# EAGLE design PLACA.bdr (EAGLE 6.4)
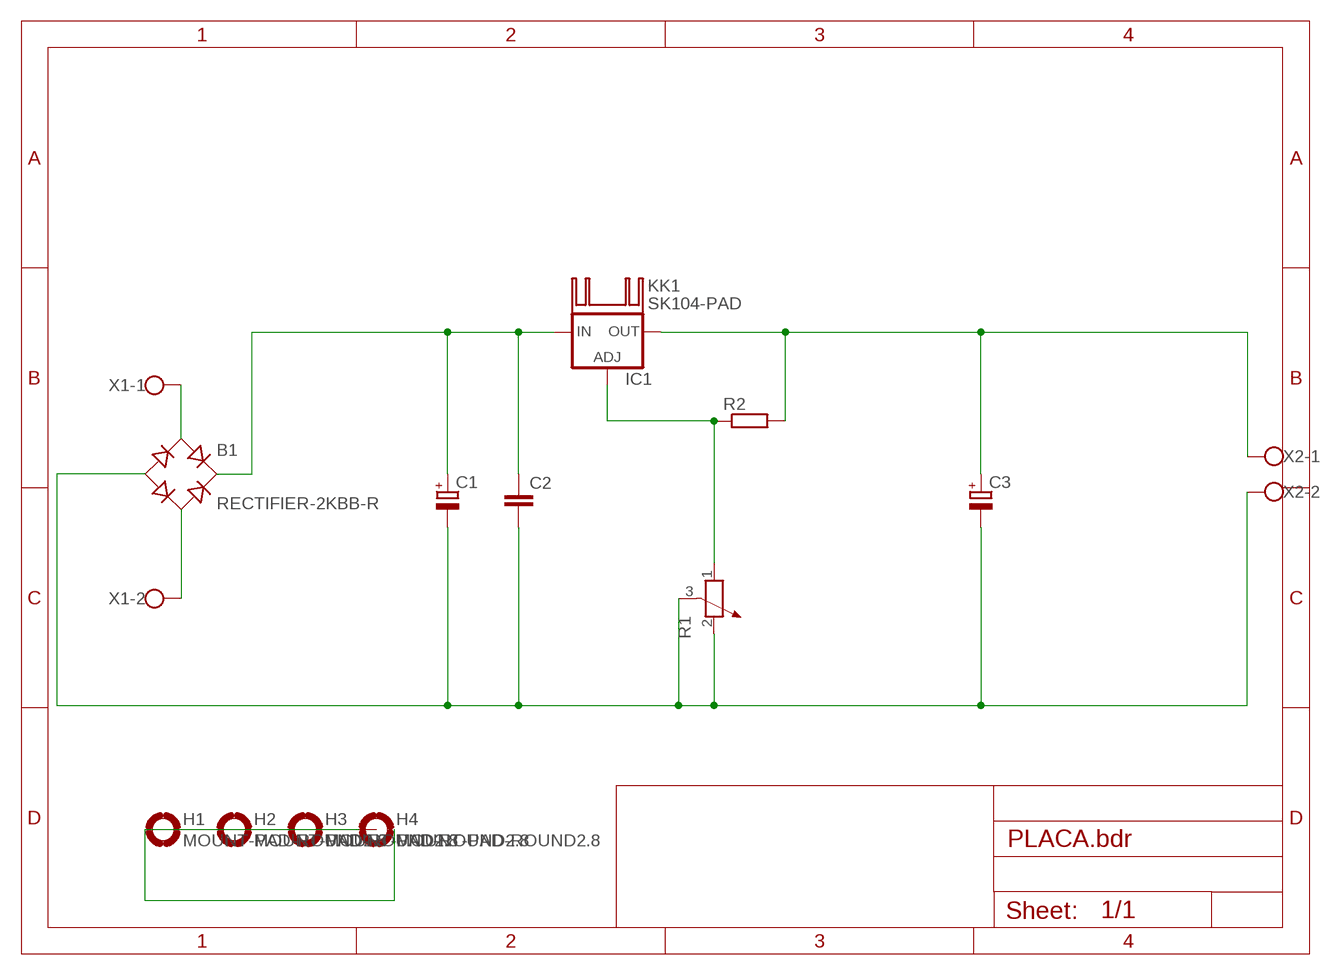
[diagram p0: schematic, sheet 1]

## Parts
B1  RECTIFIER-2KBB-R  [2KBB-R]
C1  CPOL-EUE7.5-16  [E7,5-16]
C2  C-EU050-025X075  [C050-025X075]
C3  CPOL-EUE2,5-6E  [E2,5-6E]
H1  MOUNT-PAD-ROUND2.8  [2,8-PAD]
H2  MOUNT-PAD-ROUND2.8  [2,8-PAD]
H3  MOUNT-PAD-ROUND2.8  [2,8-PAD]
H4  MOUNT-PAD-ROUND2.8  [2,8-PAD]
IC1  LM317TS  [317TS]
KK1  SK104-PAD  [SK104-PAD]
R1  POTENTIOMETER_PT-10  [PT-10]
R2  R-EU_0207/10  [0207/10]
X1  W237-102  [W237-102]
X2  W237-102  [W237-102]

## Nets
N$1: B1.AC1 X1.1
N$2: B1.AC2 X1.2
N$3: B1.- C1.- C2.2 C3.- R1.2 R1.3 X2.2
N$4: B1.+ C1.+ C2.1 IC1.3(IN)
N$5: C3.+ IC1.2(OUT) R2.2 X2.1
N$6: H1.B2,8(MOUNT) H2.B2,8(MOUNT) H3.B2,8(MOUNT) H4.B2,8(MOUNT)
N$7: IC1.1(ADJ) R1.1 R2.1
Unconnected: KK1.K1(K) KK1.K2(K)

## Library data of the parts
B1 = rectifier:RECTIFIER-: Rectifier
C1 C3 = rcl:CPOL-EU: POLARIZED CAPACITOR, European symbol
C2 = rcl:C-EU: CAPACITOR, European symbol
H1-H4 = holes:MOUNT-PAD-ROUND: MOUNTING PAD, round
IC1 = v-reg:LM317TS: VOLTAGE REGULATOR
KK1 = heatsink:SK104-PAD: HEATSINK
R1 = rcl:POTENTIOMETER_: Potentiometer
R2 = rcl:R-EU_: RESISTOR, European symbol
X1 X2 = con-wago-500:W237-102: WAGO SCREW CLAMP; MPN: 237-102; OC_FARNELL: unknown; OC_NEWARK: 70K9898

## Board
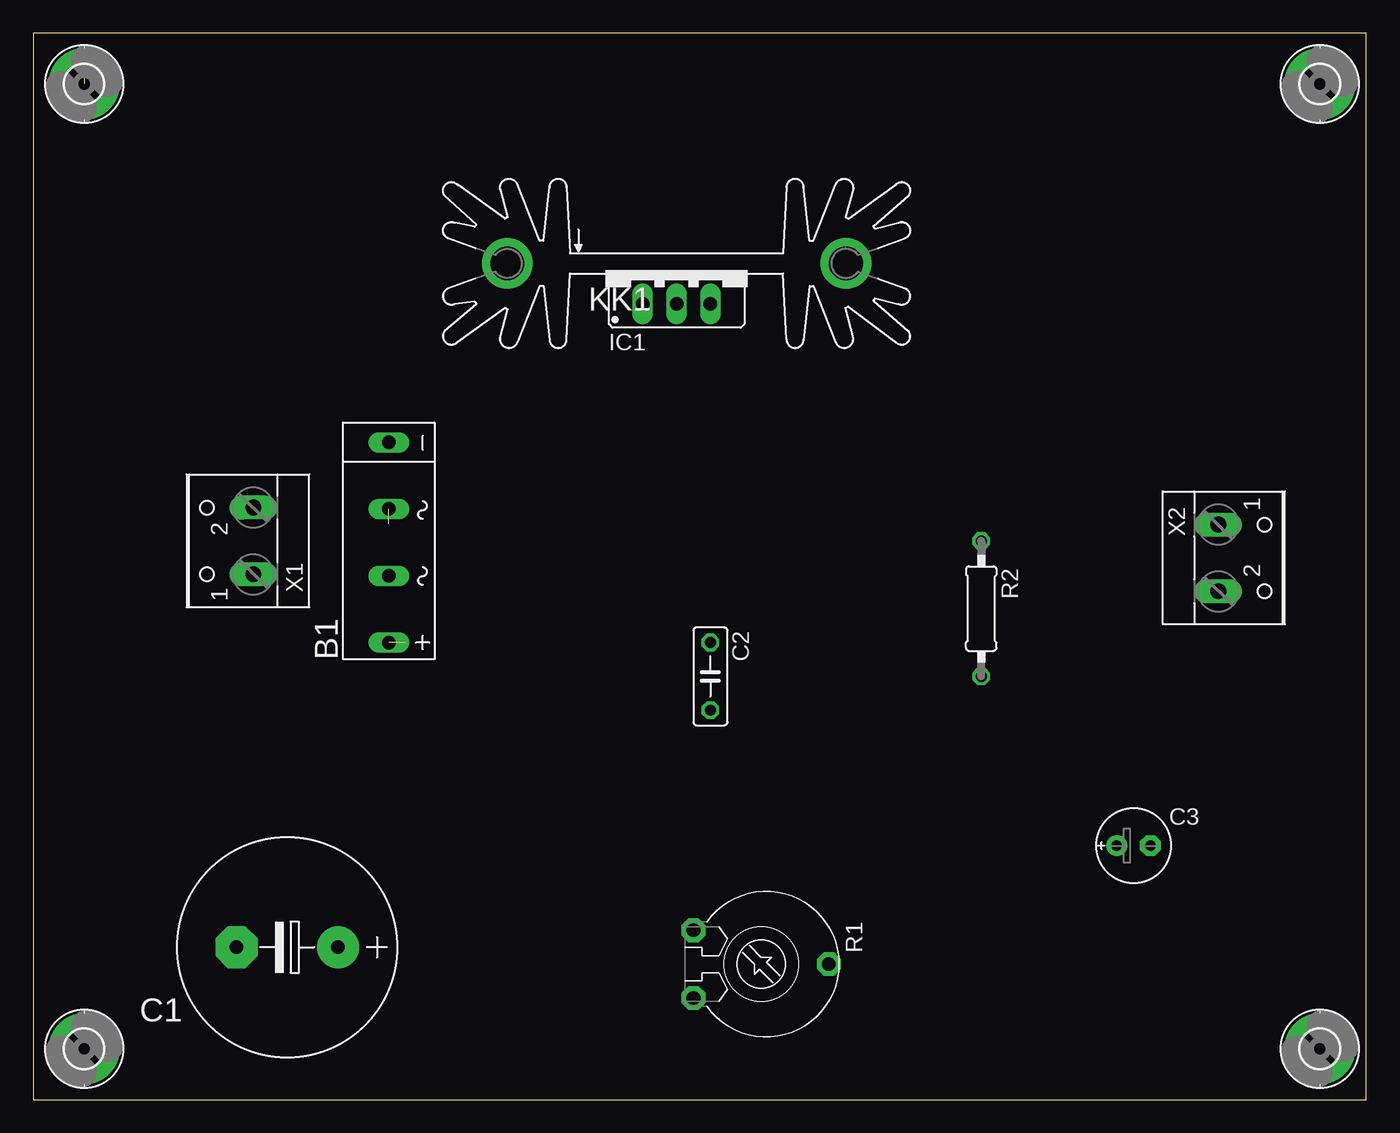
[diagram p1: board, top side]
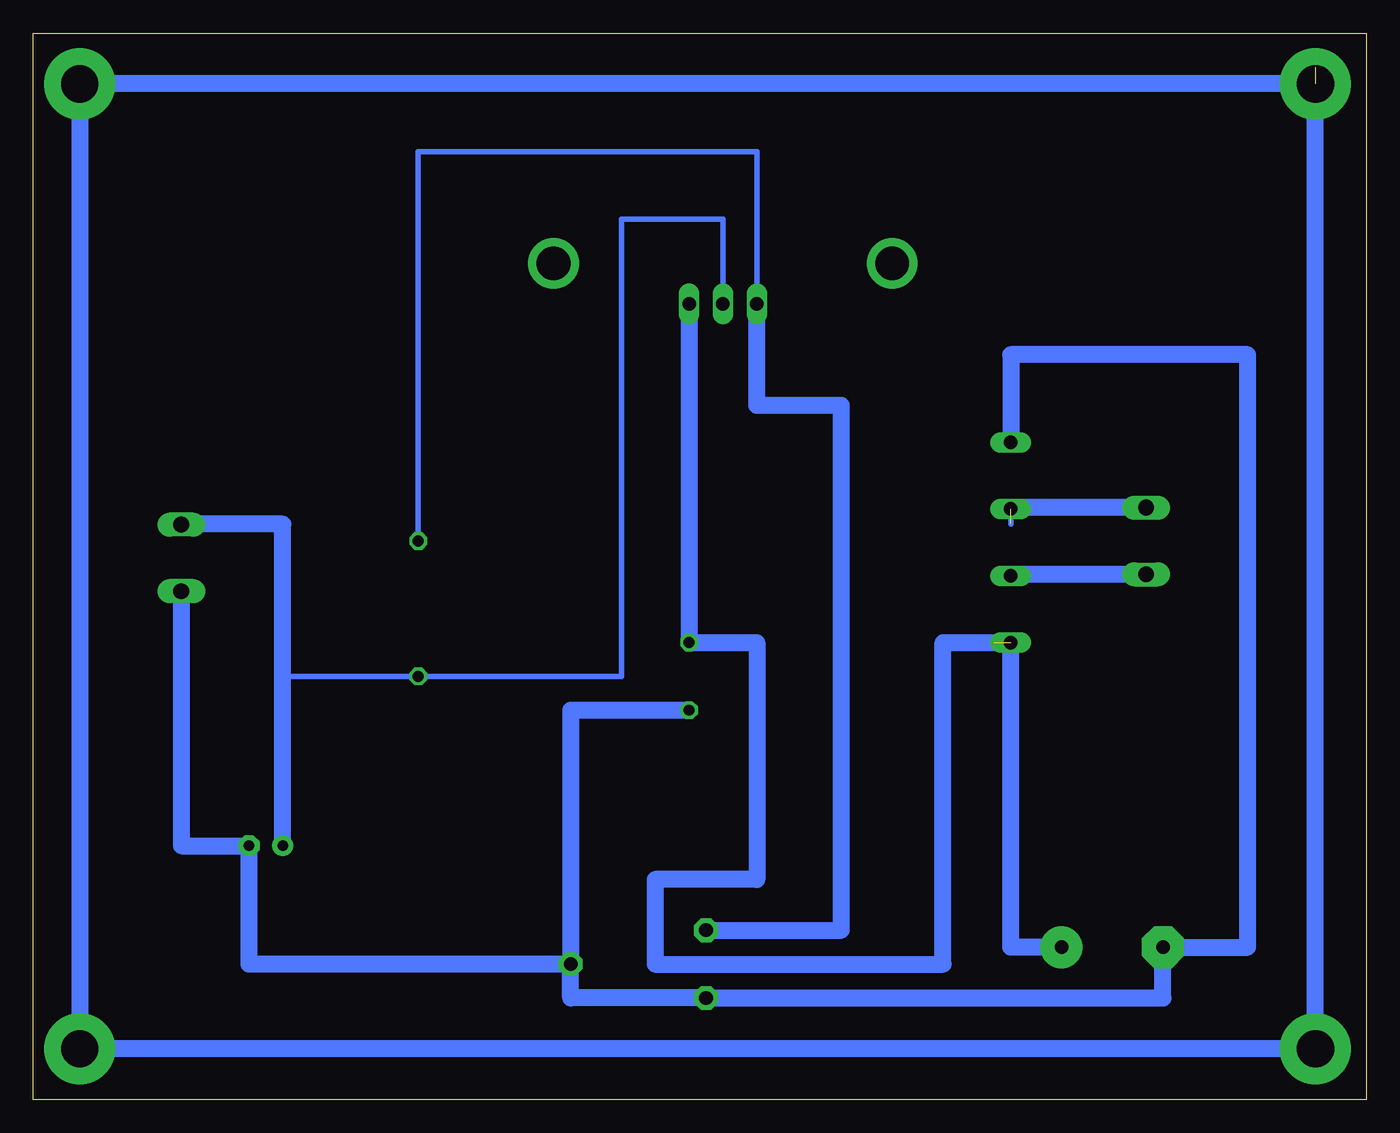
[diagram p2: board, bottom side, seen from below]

Size 100 x 80 mm. Coordinates in mm from the lower left corner, seen from the top.
Outline: 0,0 100,0 100,80 0,80 0,0
Copper layers (1*16): Top 0.035mm / dielectric 1.5mm / Bottom 0.035mm
Design rules "default": minimum track width 10mil, minimum drill 24mil, track to track 8mil, track to pad 8mil, pad to pad 8mil, via to via 8mil, smd to smd 8mil, copper to edge 40mil, drill to drill 8mil, minimum pad ring 10mil, minimum via ring 8mil, stop-mask expansion 4mil, vias tented up to drill 0mil, thermal gap 10mil

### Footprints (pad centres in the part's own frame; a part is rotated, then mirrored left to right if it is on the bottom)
2KBB-R = drill 1.016 long: + -7.62,0; - 7.391,0; AC1 -2.616,0; AC2 2.413,0
E7,5-16 = drill 1.016 pad 3.15: + -3.81,0 | drill 1.016 pad 3.15 octagon: - 3.81,0
C050-025X075 = drill 0.813 octagon: 1 -2.54,0; 2 2.54,0
E2,5-6E = drill 0.813 pad 1.575: + -1.27,0 | drill 0.813 pad 1.575 octagon: - 1.27,0
2,8-PAD = drill 2.8 pad 5.334: B2,8 0,0
317TS = drill 1.016 long: 1 -2.54,-2.54; 2 0,-2.54; 3 2.54,-2.54
SK104-PAD = drill 2.54 pad 3.81: K1 -12.7,-0.762; K2 12.7,-0.762
PT-10 = drill 1.016 pad 1.778 octagon: 1 -2.54,-5.08; 2 2.54,-5.08; 3 0,5.08
0207/10 = drill 0.813 octagon: 1 -5.08,0; 2 5.08,0
W237-102 = drill 1.194 long: 1 -2.5,-1.27; 2 2.5,-1.27

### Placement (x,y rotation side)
B1  26.67,41.91 90 top
C1  19.05,11.43 180 top
C2  50.8,31.75 270 top
C3  82.55,19.05 0 top
H1  3.81,3.81 0 top
H2  3.81,76.2 0 top
H3  96.52,76.2 0 top
H4  96.52,3.81 0 top
IC1  48.26,62.23 0 top
KK1  48.26,63.5 0 top
R1  54.61,10.16 270 top
R2  71.12,36.83 270 top
X1  15.24,41.91 90 top
X2  90.17,40.64 270 top

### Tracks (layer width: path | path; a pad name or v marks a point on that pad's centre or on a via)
N$1
  Bottom 0.406: 26.67,39.41 B1.AC1
  Bottom 1.27: X1.1 26.67,39.41
N$2  (1 unrouted)
  Bottom 0.406: 26.67,44.41 26.67,43.18
  Bottom 1.27: X1.2 26.67,44.41
N$3
  Bottom 1.27: B1.- 26.67,55.88 8.89,55.88 8.89,11.43 C1.- 15.24,7.62 R1.2 59.69,7.62 R1.3 | R1.3 83.82,10.16 C3.- 88.9,19.05 X2.2 | C2.2 59.69,29.21 R1.3
N$4  (1 unrouted)
  Bottom 1.27: C1.+ 26.67,11.43 B1.+ | IC1.3 C2.1 45.72,34.29 45.72,16.51 53.34,16.51 53.34,10.16 31.75,10.16 31.75,34.29 27.94,34.29
N$5
  Bottom 0.406: 88.9,43.18 X2.1 | 81.28,31.75 R2.2 55.88,31.75 55.88,66.04 48.26,66.04 IC1.2
  Bottom 1.27: C3.+ 81.28,31.75 81.28,43.18 88.9,43.18
N$6  (1 unrouted)
  Bottom 0.406: H2.B2,8 3.81,77.47
  Bottom 1.27: 5.08,3.81 H4.B2,8 H3.B2,8 H2.B2,8 H1.B2,8
N$7
  Bottom 0.406: IC1.1 45.72,60.96 45.72,71.12 71.12,71.12 R2.1
  Bottom 1.27: R1.1 39.37,12.7 39.37,52.07 45.72,52.07 IC1.1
